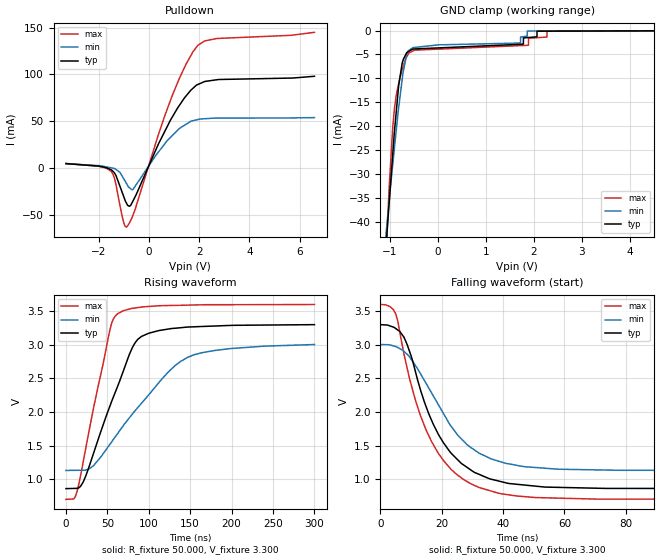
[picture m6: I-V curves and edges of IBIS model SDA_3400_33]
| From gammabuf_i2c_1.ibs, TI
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|   Input/Output open drain SDA_3400 model 3V with 3.4 MHz CLOCK
[Model]   SDA_3400_33
Model_type   I/O_open_drain
|Signals   SDA
| variable   typ   min   max
|C_comp Average
C_comp   1.2228015e-10   1.0131306e-10   1.4983527e-10
|C_comp Output Low
|C_comp   2.4268710e-10   2.0056550e-10   2.9799520e-10
|C_comp Output High
|C_comp   1.8731950e-12   2.0606150e-12   1.6753480e-12
Vinl = 0.99
Vinh = 2.31
Vmeas = 1.65
Vref = 1.65
Cref = 15pF
Rref = 50
[Voltage Range]   3.3   3   3.6
[Temperature Range]   27   85   -40
[Pullup Reference]   3.3   3   3.6
[Pulldown Reference]   0   0   0
[Power Clamp Reference]   3.3   3   3.6
[GND Clamp Reference]   -0   0   -0
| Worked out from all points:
|   slope of the pulldown table from 0 to 0.495 V, typ, clamps not added: 16.9 ohm
|   falling waveform, R_fixture 50.000, V_fixture 3.300: 20-80 % time 13.7ns typ, 16.2ns min, 13.5ns max; typ from 3.3 V to 0.859 V
|   rising waveform, R_fixture 50.000, V_fixture 3.300: 20-80 % time 42.9ns typ, 74.2ns min, 28.5ns max; typ from 0.859 V to 3.3 V
[Pulldown]
|   Voltage   I(typ)   I(min)   I(max)
-3.3V     4.939mA    4.943mA    5.153mA
-1.512V   -1.485mA   561.9uA    -2.965mA
-1.368V   -5.11mA    -176.2uA   -10.69mA
-1.031V   -27.95mA   -9.801mA   -54.91mA
-890.7mV  -37.21mA   -16.19mA   -62.75mA
-774.6mV  -40.51mA   -20.72mA   -58.23mA
-624.8mV  -34.41mA   -22.32mA   -49.45mA
924.3mV   54.25mA    34.63mA    77.01mA
1.481V    77.06mA    46.91mA    111mA
1.947V    89.26mA    51.9mA     131mA
2.694V    94.28mA    53.44mA    138.3mA
6.59V     98.03mA    54mA       144.9mA
[GND Clamp]
|   Voltage   I(typ)   I(min)   I(max)
-3.3V     -394mA     -291.8mA   -588.8mA
-1.129V   -52.11mA   -47.38mA   -56.46mA
-1.049V   -40.26mA   -38.9mA    -39.54mA
-943.4mV  -25.89mA   -28.03mA   -20.33mA
-871.1mV  -17.12mA   -20.96mA   -13.64mA
-739.4mV  -6.584mA   -9.68mA    -7.961mA
-641.8mV  -4.561mA   -4.722mA   -5.324mA
-519.4mV  -3.859mA   -3.561mA   -4.252mA
1.719V    -2.875mA   -2.612mA   -3.149mA
1.881V    -1.461mA   -101.5uA   -3.079mA
2.279V    -131.5uA   -92.93uA   -154.9uA
6.59V     0A         0A         0A
[POWER Clamp]
|   No ESD cells to VDD
|   Voltage   I(typ)   I(min)   I(max)
-3.3V     0A         0A         0A
0V        0A         0A         0A
6.6V      0A         0A         0A
[Ramp]
R_load = 50
|   typ   min   max
dV/dt_r   1.46456/4.27845e-008   1.13827/7.40993e-008   1.74023/2.85031e-008
dV/dt_f   1.46456/1.36572e-008   1.13827/1.6187e-008   1.74023/1.35275e-008
[Falling Waveform]
R_fixture = 50.000
V_fixture = 3.300
V_fixture_min = 3.000
V_fixture_max = 3.600
C_fixture = 0.000
|  time   V(typ)   V(min)   V(max)
0s        3.3V       3.004V     3.6V
4.975ns   3.243V     2.975V     3.462V
7.704ns   3.11V      2.902V     2.859V
13.06ns   2.33V      2.57V      1.947V
18.57ns   1.698V     2.136V     1.409V
23.12ns   1.384V     1.784V     1.144V
28.22ns   1.177V     1.516V     965.5mV
38.43ns   973.5mV    1.269V     792.1mV
77.77ns   862mV      1.132V     703mV
300ns     859.1mV    1.13V      699.6mV
[Rising Waveform]
R_fixture = 50.000
V_fixture = 3.300
V_fixture_min = 3.000
V_fixture_max = 3.600
C_fixture = 0.000
|  time   V(typ)   V(min)   V(max)
0s        859.1mV    1.13V      699.6mV
9.301ns   861.8mV    1.131V     704mV
13.25ns   862.9mV    1.132V     810.5mV
23.8ns    1.044V     1.134V     1.452V
53.1ns    2.089V     1.519V     3.225V
62.28ns   2.379V     1.677V     3.462V
86.55ns   3.079V     2.064V     3.554V
123.7ns   3.235V     2.597V     3.585V
147.3ns   3.264V     2.816V     3.591V
300ns     3.3V       3.004V     3.6V
